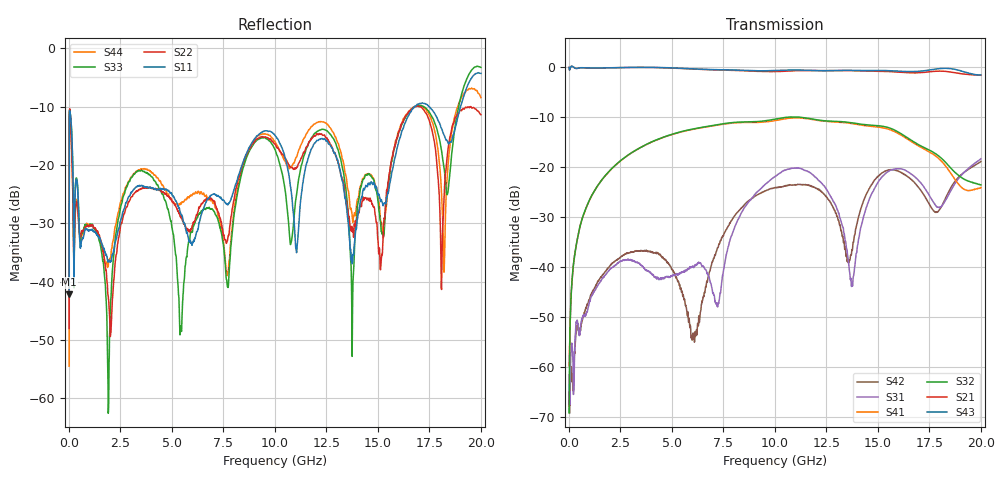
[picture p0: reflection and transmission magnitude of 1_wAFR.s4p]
!Keysight Technologies,N5225A,MY51451420,A.10.40.12
!Date: Tuesday, October 13, 2015 10:13:18
!Correction: S11(Full 4 Port(1,2,3,4))
!S12(Full 4 Port(1,2,3,4))
!S13(Full 4 Port(1,2,3,4))
!S14(Full 4 Port(1,2,3,4))
!S21(Full 4 Port(1,2,3,4))
!S22(Full 4 Port(1,2,3,4))
!S23(Full 4 Port(1,2,3,4))
!S24(Full 4 Port(1,2,3,4))
!S31(Full 4 Port(1,2,3,4))
!S32(Full 4 Port(1,2,3,4))
!S33(Full 4 Port(1,2,3,4))
!S34(Full 4 Port(1,2,3,4))
!S41(Full 4 Port(1,2,3,4))
!S42(Full 4 Port(1,2,3,4))
!S43(Full 4 Port(1,2,3,4))
!S44(Full 4 Port(1,2,3,4))
!S4P File: Measurements: <S11,S12,S13,S14>,
!<S21,S22,S23,S24>,
!<S31,S32,S33,S34>,
!<S41,S42,S43,S44>:
# Hz S  dB  R 50
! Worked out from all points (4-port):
!   2000 points, 10 MHz to 20 GHz, reference 50 ohm
!   strongest paths, dB at 10 MHz, 5.01 GHz, 10.01 GHz, 15.01 GHz, 20 GHz:
!     S43: -0.1, -0.2, -0.7, -0.7, -1.5
!     S21: 0.0, -0.2, -0.9, -0.8, -1.6
!     S32: -69.3, -13.5, -10.4, -11.7, -23.6
!     S41: -59.8, -13.5, -10.7, -12.0, -24.1
!     S31: -61.6, -41.8, -21.9, -23.0, -18.4
!     S42: -67.9, -40.6, -24.1, -21.8, -18.9
!   lowest |S11| = -42.2 dB at 10 MHz (marker M1), VSWR 1.02, Z = 50.7 - j0.341 ohm
!   |S11| at or under -10 dB: start of sweep to 16.77 GHz; 17.5 GHz to 19.01 GHz (1.503 GHz wide, 8.23 % of centre)
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1e7  -42.16 -25.5  -0.03 0.3  -61.99 107.3  -59.01 82.0
     -0.04 0.5  -48.03 162.3  -63.86 95.3  -78.86 22.3
     -61.63 -73.2  -69.25 -159.4  -40.45 -16.0  -0.07 0.6
     -59.84 95.9  -67.85 -75.8  -0.07 0.2  -54.48 -161.4
1.92e9  -36.51 111.1  -0.15 6.7  -40.90 50.4  -21.04 96.7
        -0.16 6.8  -43.03 151.3  -21.00 96.7  -40.31 126.9
        -40.89 50.3  -21.01 96.7  -62.19 -53.7  -0.17 6.9
        -21.05 96.8  -40.21 127.4  -0.15 6.9  -36.81 -144.6
4e9  -23.92 -162.4  -0.06 19.6  -41.34 -51.1  -15.04 109.9
     -0.06 19.7  -23.94 24.2  -15.00 109.8  -37.04 127.1
     -41.38 -50.6  -15.02 109.9  -21.98 -162.6  -0.07 20.2
     -15.03 109.9  -37.06 127.7  -0.05 20.2  -21.27 26.3
5.43e9  -28.27 -126.5  -0.25 28.7  -41.18 -145.1  -13.00 119.0
        -0.26 28.9  -28.68 85.8  -12.95 119.1  -44.16 107.1
        -41.27 -145.3  -12.96 119.1  -47.81 102.3  -0.24 29.4
        -13.01 119.2  -44.22 106.8  -0.23 29.4  -26.69 132.0
1.246e10  -15.70 -147.2  -0.70 59.2  -24.19 -41.5  -10.87 149.0
          -0.71 59.6  -15.24 87.1  -10.75 149.0  -25.79 -147.7
          -24.19 -41.0  -10.77 148.9  -14.00 -161.2  -0.74 60.0
          -10.87 149.5  -25.82 -147.8  -0.72 60.2  -12.78 100.5
1.376e10  -36.91 -74.4  -0.72 65.2  -43.58 -27.2  -11.32 155.9
          -0.72 65.6  -31.46 -157.0  -11.17 156.5  -36.76 -43.9
          -43.55 -26.9  -11.18 156.3  -47.84 66.5  -0.65 66.4
          -11.32 156.3  -36.69 -44.0  -0.65 66.6  -29.17 -146.6
2e10  -4.27 -122.1  -1.60 93.3  -18.35 -109.7  -24.17 -131.6
      -1.60 93.8  -11.36 -175.2  -23.57 -139.4  -18.91 127.7
      -18.37 -109.5  -23.59 -139.8  -3.25 -116.5  -1.56 92.8
      -24.15 -131.1  -18.90 127.6  -1.55 93.1  -8.42 168.1
